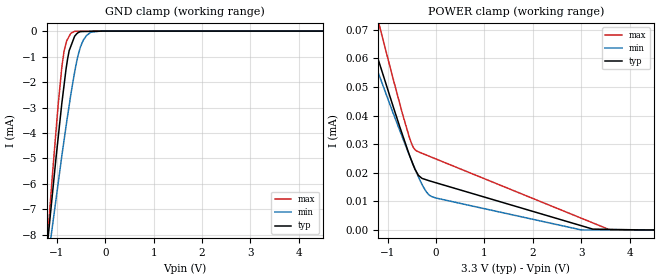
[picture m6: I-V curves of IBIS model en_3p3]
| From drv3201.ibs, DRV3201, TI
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|   en_3p3 Model
[Model]   en_3p3
Model_type   Input
Vinl = 0.99
Vinh = 2.31
|   typ   min   max
|   (nom PVT)   (fast PVT)   (slow PVT)
C_comp   4.837e-13   4.556e-13   5.160e-13
| Where nom  PVT is Nominal Process, 3.3V, 27C
|   Fast PVT is Strong Process,  3.6V, -40C
|   Slow PVT is Weak Process,   3V, 150C
[Voltage Range]   3.3   3   3.6
[Temperature Range]   27   150   -40
[Power Clamp Reference]   3.3   3   3.6
[GND Clamp Reference]   0   0   0
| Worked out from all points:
|   GND clamp passes 1 mA (typ) near -0.77 V on its own axis
[GND Clamp]
|   Voltage   I(typ)   I(min)   I(max)
-3.3V     -51.88mA   -41.42mA   -64.02mA
-1.181V   -8.102mA   -8.925mA   -7.87mA
-1.094V   -6.441mA   -7.691mA   -5.702mA
-975.6mV  -4.226mA   -6.005mA   -2.945mA
-896.4mV  -2.818mA   -4.881mA   -1.396mA
-849.6mV  -2.095mA   -4.261mA   -766.3uA
-745.8mV  -768uA     -2.917mA   -203.4uA
-633.6mV  -205.1uA   -1.62mA    -9.813uA
-561mV    -59.98uA   -948.6uA   -5.723uA
-456mV    -16.51uA   -362.6uA   -3.147uA
-285mV    -10.28uA   -39.12uA   -1.965uA
6.6V      0A         0A         0A
[POWER Clamp]
|   Voltage   I(typ)   I(min)   I(max)
-3.3V     174.7uA    153.2uA    214.6uA
-1.71V    87.47uA    78.65uA    107.4uA
-1.238V   61.92uA    56.99uA    75.88uA
-897.6mV  43.75uA    41.33uA    53.51uA
-687.6mV  32.97uA    32.07uA    40.22uA
-475.2mV  22.83uA    22.97uA    29.05uA
-366.3mV  19.12uA    18.66uA    27.37uA
-204mV    17.56uA    13.41uA    26.22uA
-84mV     16.92uA    11.63uA    25.4uA
2.997V    1.515uA    13.07nA    4.157uA
3.596V    198.8nA    0A         24.81nA
6.6V      0A         0A         0A
